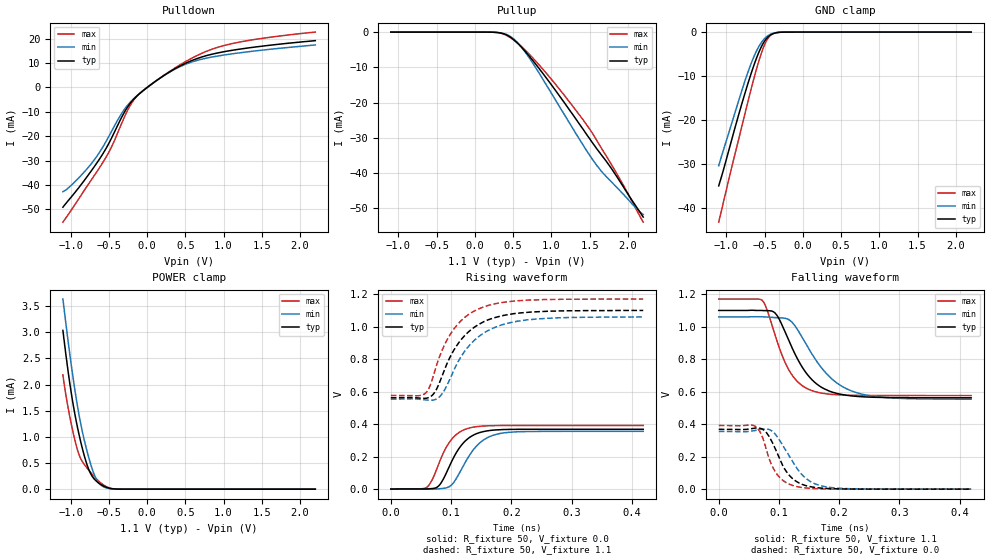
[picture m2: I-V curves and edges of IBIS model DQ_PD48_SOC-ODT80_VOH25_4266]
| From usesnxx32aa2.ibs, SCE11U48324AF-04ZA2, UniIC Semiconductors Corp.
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| DQ_PD48_SOC-ODT80_VOH25_4266
| (48 Ohm Pulldown, 80 Ohm System ODT Setting, VOH=VDDQ/2.5, 3200-4266Mbps)
[Model]   DQ_PD48_SOC-ODT80_VOH25_4266
Model_type   I/O
Vinl = 160.000mV
Vinh = 280.000mV
Vmeas = 220.000mV
Vref = 0.0mV
Cref = 0.0pF
Rref = 80.000Ohm
|   typ   min   max
|C_comp   0.797pF   0.747pF   0.847pF
C_comp_pullup   0.3985pF   0.3735pF   0.4235pF
C_comp_pulldown   0.3985pF   0.3735pF   0.4235pF
| Note: C_comp changes when the ODT circuit is enabled.
[Model Spec]
| Input threshold voltage corners
Vinl   0.1600V   0.1520V   0.1740V
Vinh   0.2800V   0.2720V   0.2940V
| Measurement voltage corners
Vmeas   0.2200V   0.2120V   0.2340V
| Timing spec test load voltage corners
Vref   0.0000V   0.0000V   0.0000V
| Dynamic Overshoot Parameters from LPDDR4 Specification
D_overshoot_ampl_h   0.30   NA   NA
D_overshoot_ampl_l   0.30   NA   NA
D_overshoot_area_h   0.1n   NA   NA
D_overshoot_area_l   0.1n   NA   NA
[Receiver Thresholds]
Vth   = 0.2200V
Vth_min  = 0.2167V
Vth_max  = 0.2233V
Vinh_ac  = 0.060V
Vinh_dc  = 0.060V
Vinl_ac  = -0.060V
Vinl_dc  = -0.060V
Tslew_ac = 5.000ns |Not specified, so set to high value
Threshold_sensitivity = 0.2000
Reference_supply Pullup_ref
[Voltage Range]   1.1000V   1.0600V   1.1700V
[Pullup Reference]   1.1000V   1.0600V   1.1700V
| Junction Temperature (Ambient temp is 35C typ 95C min -40C max)
[Temperature Range]   50.0   110.0   -40.0
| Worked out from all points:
|   slope of the pulldown table from 0 to 0.165 V, typ, clamps not added: 43.8 ohm
|   slope of the pullup table from 0 to 0.165 V, typ, clamps not added: 17.1 kohm
|   GND clamp passes 1 mA (typ) near -0.45 V on its own axis
|   POWER clamp passes 1 mA (typ) near -0.88 V on its own axis
|   rising waveform, R_fixture 50, V_fixture 0.0: 20-80 % time 34.2ps typ, 37.9ps min, 31.2ps max; typ from 0.001 V to 0.369 V
|   falling waveform, R_fixture 50, V_fixture 1.1: 20-80 % time 48.4ps typ, 61ps min, 38.3ps max; typ from 1.1 V to 0.563 V
|   rising waveform, R_fixture 50, V_fixture 1.1: 20-80 % time 54.7ps typ, 58.1ps min, 50.6ps max; typ from 0.562 V to 1.1 V
|   falling waveform, R_fixture 50, V_fixture 0.0: 20-80 % time 32ps typ, 39.4ps min, 26.4ps max; typ from 0.369 V to 0.001 V
[Pulldown]
|   Voltage   I(typ)   I(min)   I(max)
-1.1V     -49.08mA   -42.7mA    -55.23mA
-776.6mV  -36.24mA   -33.06mA   -40.12mA
-638mV    -30.11mA   -27.36mA   -33.66mA
-522.5mV  -24.24mA   -21.38mA   -27.85mA
-334.4mV  -12.38mA   -10.76mA   -14.9mA
-195.8mV  -5.557mA   -5.256mA   -6.129mA
-116.6mV  -3.032mA   -2.973mA   -3.076mA
45.1mV    1.049mA    1.046mA    1.047mA
474.1mV   9.491mA    9.153mA    10.08mA
896.5mV   13.98mA    12.75mA    16.19mA
1.335V    16.27mA    14.7mA     19.33mA
2.2V      19.2mA     17.45mA    22.72mA
[GND Clamp]
|   Voltage   I(typ)   I(min)   I(max)
-1.1V     -34.89mA   -30.33mA   -43.14mA
-944.9mV  -25.34mA   -21.52mA   -31.72mA
-799.7mV  -16.38mA   -13.37mA   -21.53mA
-733.7mV  -12.54mA   -9.877mA   -16.88mA
-667.7mV  -8.943mA   -6.741mA   -12.35mA
-591.8mV  -5.275mA   -3.797mA   -7.53mA
-522.5mV  -2.673mA   -1.907mA   -3.826mA
-469.7mV  -1.361mA   -988.9uA   -1.791mA
-416.9mV  -597.6uA   -442.1uA   -665.5uA
-354.2mV  -179.1uA   -135.4uA   -160.3uA
-255.2mV  -14.69uA   -13.18uA   -8.81uA
2.2V      0A         0A         0A
[Pullup]
|   Voltage   I(typ)   I(min)   I(max)
-1.1V     4.112uA    7.441uA    1.363uA
259.6mV   -61.43uA   -59.36uA   -61.49uA
391.6mV   -603.2uA   -502uA     -719.1uA
507.1mV   -2.161mA   -1.951mA   -2.252mA
616mV     -4.459mA   -4.485mA   -4.266mA
748mV     -7.819mA   -8.539mA   -7.138mA
1.032V    -15.9mA    -18.5mA    -14.23mA
1.444V    -28.51mA   -33.07mA   -25.79mA
1.655V    -34.88mA   -39.5mA    -32.99mA
1.801V    -39.21mA   -42.84mA   -38.16mA
1.943V    -43.96mA   -46.05mA   -43.51mA
2.2V      -52.46mA   -51.74mA   -53.91mA
[POWER Clamp]
|   Voltage   I(typ)   I(min)   I(max)
-1.1V     3.036mA    3.636mA    2.186mA
-1.044V   2.383mA    2.969mA    1.654mA
-977.9mV  1.724mA    2.242mA    1.161mA
-908.6mV  1.178mA    1.583mA    748.4uA
-852.5mV  818.5uA    1.149mA    543.8uA
-776.6mV  434.3uA    683.6uA    390.2uA
-710.6mV  232.2uA    359.3uA    273.1uA
-651.2mV  138.6uA    162.3uA    181.2uA
-591.8mV  78uA       64.8uA     105.5uA
-489.5mV  17.77uA    10.83uA    22.44uA
-380.6mV  1.61uA     1.14uA     1.336uA
2.2V      0A         0A         0A
[Ramp]
|   typ   min   max
| 20% - 80%
dV/dt_r   220.81m/34.25p   213.14m/37.95p   234.88m/31.16p
dV/dt_f   322.45m/48.44p   303.64m/60.98p   356.23m/38.27p
| 25% - 75%
|dV/dt_r   184.01m/27.26p   177.62m/30.23p   195.73m/24.71p
|dV/dt_f   268.71m/38.64p   253.04m/48.62p   296.86m/30.47p
R_load = 50
[Rising Waveform]
R_fixture = 50
V_fixture = 0.0
|   Time   V(typ)   V(min)   V(max)
0s        640uV      516.9uV    470.5uV
58ps      699.9uV    85.29uV    7.425mV
67ps      2.747mV    -292.1uV   46.13mV
77ps      12.23mV    1.048mV    131.1mV
101ps     170.4mV    26.22mV    306.9mV
115ps     259.7mV    106.2mV    352.8mV
130ps     316.3mV    205.1mV    375.9mV
155ps     355.2mV    305.2mV    388.8mV
188ps     366.9mV    346.4mV    391.6mV
419ps     368.7mV    355.8mV    391.9mV
[Falling Waveform]
R_fixture   = 50
V_fixture   = 1.1
V_fixture_min = 1.06
V_fixture_max = 1.17
|   Time   V(typ)   V(min)   V(max)
0s        1.1V       1.06V      1.17V
72ps      1.1V       1.061V     1.163V
81ps      1.099V     1.059V     1.095V
95ps      1.078V     1.056V     931.4mV
115ps     926.7mV    1.046V     743.5mV
133ps     786.4mV    968.9mV    654.1mV
153ps     680.5mV    842.6mV    608.9mV
188ps     598mV      678.1mV    583.5mV
231ps     570.6mV    591.7mV    577.4mV
419ps     562.6mV    553.9mV    576.3mV
[Rising Waveform]
R_fixture   = 50
V_fixture   = 1.1
V_fixture_min = 1.06
V_fixture_max = 1.17
|   Time   V(typ)   V(min)   V(max)
0s        562.5mV    553.6mV    576.3mV
57ps      558.7mV    549.1mV    589.3mV
65ps      567.3mV    546.5mV    634.9mV
78ps      631.2mV    559.5mV    785.8mV
93ps      770.5mV    636.8mV    916.2mV
111ps     892.1mV    779.5mV    1.015V
130ps     971.5mV    883mV      1.077V
152ps     1.026V     955.2mV    1.119V
226ps     1.088V     1.042V     1.163V
419ps     1.1V       1.06V      1.17V
[Falling Waveform]
R_fixture = 50
V_fixture = 0.0
|   Time   V(typ)   V(min)   V(max)
0s        368.8mV    355.9mV    392mV
58ps      375.2mV    359.8mV    391.7mV
74ps      366.4mV    371.1mV    306mV
85ps      315.6mV    365.5mV    175mV
95ps      239.6mV    333.4mV    101.1mV
110ps     121.7mV    247.1mV    45.17mV
128ps     50.08mV    138.7mV    17.66mV
151ps     16.58mV    50.17mV    5.647mV
184ps     3.957mV    11.51mV    1.449mV
419ps     686.6uV    583.4uV    490.7uV
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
